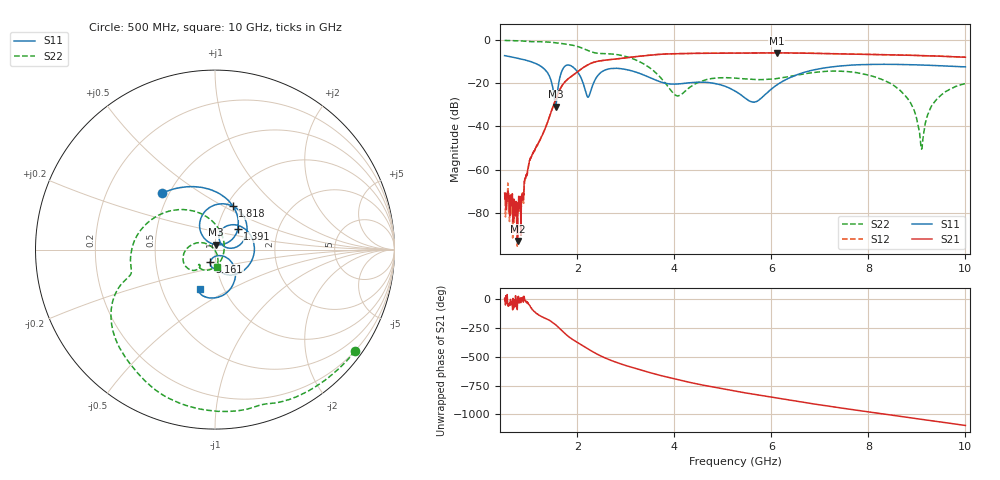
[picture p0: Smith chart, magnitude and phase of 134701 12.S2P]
!  2-Port S-parameters saved by WinCal
! VAR MeasName=S-Parameters (CALIBRATED_DATA) read from VNA (N5242A)
! VAR MeasDate=2013-7-3 16:29:09
! VAR NAME=134701 12
! VAR FILENAME=134701 12.S2P
! VAR DATE=2013-7-3 16:29:09
! VAR PHYS_PORTS=1,2
# Hz S MA R 50
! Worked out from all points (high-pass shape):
!   1601 points, 500 MHz to 10 GHz, reference 50 ohm
!   highest |S21| = -6.07 dB at 6.111 GHz (marker M1); lowest = -92.8 dB at 767.2 MHz (marker M2)
!   |S21| within 3 dB of the highest: 2.715 GHz to end of sweep
!   lowest |S11| = -30.9 dB at 1.551 GHz (marker M3), VSWR 1.06, Z = 50.5 + j2.83 ohm
!   |S11| at or under -10 dB: 1.027 GHz to end of sweep
!   |S22| runs from -50.5 to -0.3 dB; largest |S21 - S12| = 0.0027
!   S11 on the Smith chart (normalised r, x): 500 MHz: 0.46, +0.36; 1.391 GHz: 1.25, +0.29; 1.818 GHz: 1.07, +0.56; 5.161 GHz: 0.94, -0.13; 10 GHz: 0.77, -0.36
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5e8  0.4305 133.0  0.0002891 2.4  0.0002422 -22.9  0.963 -35.9
7.671875e8  0.3753 110.7  2.283e-05 -2.8  0.0001471 18.8  0.9456 -54.9
1.04625e9  0.3109 84.8  0.001922 -78.4  0.001915 -75.5  0.9026 -73.7
1.390625e9  0.1699 41.7  0.01298 -176.9  0.01286 -178.0  0.8867 -98.5
1.550938e9  0.02848 79.2  0.04165 137.4  0.04155 137.2  0.8564 -111.0
1.681562e9  0.191 114.5  0.08657 85.9  0.08634 85.8  0.8169 -120.9
1.818125e9  0.2614 67.9  0.1276 34.1  0.1272 34.0  0.7762 -131.0
2.085312e9  0.1246 7.6  0.2137 -39.0  0.2132 -39.0  0.651 -151.9
2.227812e9  0.04769 46.0  0.2686 -75.2  0.2681 -75.1  0.5581 -159.6
2.797812e9  0.2195 0.3  0.36 171.6  0.3597 171.7  0.4573 176.3
3.670625e9  0.1112 -79.3  0.4588 62.0  0.4584 62.0  0.1519 93.0
4.068438e9  0.09555 -78.4  0.4794 20.6  0.4792 20.5  0.05047 -6.7
5.160938e9  0.07429 -110.9  0.4911 -71.5  0.4916 -71.5  0.1324 -132.2
5.25e9  0.06567 -111.5  0.4921 -78.1  0.4921 -78.2  0.1305 -134.2
5.65375e9  0.0364 -71.2  0.4949 -107.3  0.4955 -107.3  0.1211 -136.6
6.110938e9  0.09034 -34.6  0.4973 -138.9  0.4969 -138.9  0.1274 -131.5
6.835312e9  0.1967 -55.5  0.4879 173.1  0.4881 173.1  0.1734 -138.5
8.420625e9  0.2707 -98.5  0.4499 77.0  0.4498 76.9  0.103 158.3
8.865938e9  0.2655 -105.1  0.4369 50.8  0.4382 50.6  0.03533 141.0
9.0975e9  0.2612 -107.7  0.4311 37.1  0.4308 37.1  0.00299 -136.9
9.364688e9  0.2545 -109.9  0.4207 21.5  0.4224 21.4  0.03711 -68.3
1e10  0.2368 -110.9  0.3954 -15.8  0.3963 -15.9  0.0973 -85.0
